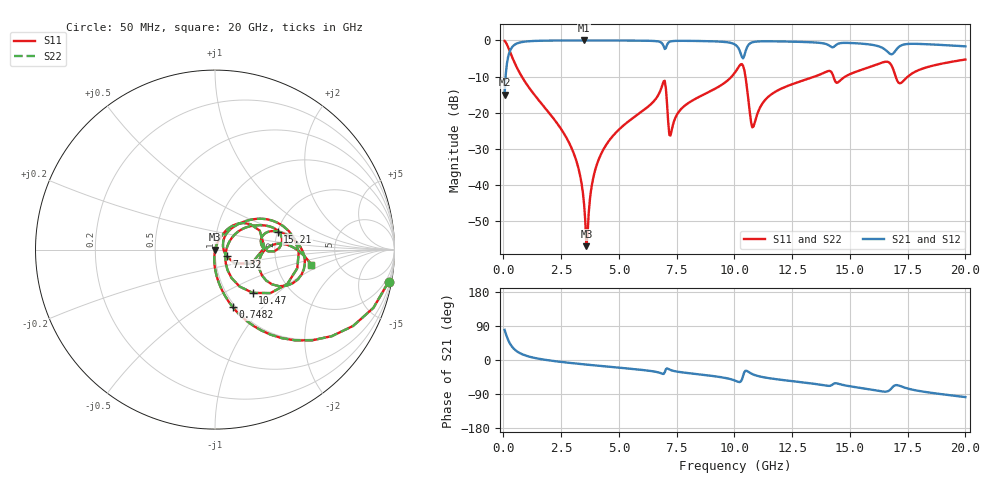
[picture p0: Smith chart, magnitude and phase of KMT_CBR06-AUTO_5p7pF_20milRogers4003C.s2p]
! Data measured by Modelithics Inc. support@modelithics.com 813-866-6335
! KEMET CBR06-AUTO 5.7pF, Pad Width= 0.851mm, Pad Length= 0.64mm, Pad Gap= 0.62mm, 20mil Rogers 4003C substrate Data, January 2022
# hz S ma R 50
! 2 Port Network Data from SP1.SP block
! freq  magS11  angS11  magS21  angS21  magS12  angS12  magS22  angS22
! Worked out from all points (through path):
!   401 points, 50 MHz to 20 GHz, reference 50 ohm
!   highest |S21| = -0.01 dB at 3.491 GHz (marker M1); lowest = -15.0 dB at 50 MHz (marker M2)
!   group delay of S21, straight-line fit = 15.2 ps
!   lowest |S11| = -57.0 dB at 3.591 GHz (marker M3), VSWR 1.00, Z = 50.1 - j0.0907 ohm
!   |S11| at or under -10 dB: 792.2 MHz to 9.883 GHz (9.091 GHz wide, 170 % of centre); 10.48 GHz to 13.48 GHz (3.003 GHz wide, 25.1 % of centre); 16.98 GHz to 17.51 GHz (531.9 MHz wide, 3.08 % of centre)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
!   |S22| runs from -57.0 to -0.1 dB; largest |S21 - S12| = 0
!   S11 on the Smith chart (normalised r, x): 50 MHz: 1, -11; 748.2 MHz: 0.97, -0.70; 7.132 GHz: 1.13, -0.09; 10.47 GHz: 1.32, -0.71; 15.21 GHz: 2.00, +0.46; 20 GHz: 3.17, -0.77
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5e7  0.984 -10.4  0.1777 79.6  0.1777 79.6  0.984 -10.4
2.99375e8  0.6763 -48.4  0.736 41.5  0.736 41.5  0.6763 -48.4
7.4825e8  0.3343 -72.9  0.9418 17.0  0.9418 17.0  0.3343 -72.9
2.74325e9  0.04386 -95.3  0.9978 -6.8  0.9978 -6.8  0.04386 -95.3
3.391625e9  0.00997 -93.9  0.9986 -10.9  0.9986 -10.9  0.00997 -93.9
3.491375e9  0.005367 -88.3  0.9986 -11.5  0.9986 -11.5  0.005367 -88.3
3.591125e9  0.001412 -39.9  0.9986 -12.1  0.9986 -12.1  0.001412 -39.9
3.94025e9  0.01472 70.7  0.9984 -14.2  0.9984 -14.2  0.01472 70.7
4.33925e9  0.03133 71.0  0.9979 -16.5  0.9979 -16.5  0.03133 71.0
6.73325e9  0.1827 50.5  0.9629 -33.1  0.9629 -33.1  0.1827 50.5
6.93275e9  0.2709 23.0  0.8362 -36.9  0.8362 -36.9  0.2709 23.0
7.13225e9  0.07484 -30.5  0.9254 -23.5  0.9254 -23.5  0.07484 -30.5
7.281875e9  0.05665 38.3  0.9751 -27.4  0.9751 -27.4  0.05665 38.3
1.0025e10  0.3598 26.5  0.8769 -54.3  0.8769 -54.3  0.3598 26.5
1.047388e10  0.3203 -48.9  0.6932 -28.6  0.6932 -28.6  0.3203 -48.9
1.0823e10  0.06373 1.5  0.9499 -38.4  0.9499 -38.4  0.06373 1.5
1.152125e10  0.1715 37.7  0.9727 -48.2  0.9727 -48.2  0.1715 37.7
1.336662e10  0.3071 26.0  0.9411 -62.1  0.9411 -62.1  0.3071 26.0
1.5212e10  0.363 16.0  0.915 -71.4  0.915 -71.4  0.363 16.0
1.670825e10  0.4914 -19.5  0.6619 -80.2  0.6619 -80.2  0.4914 -19.5
1.7207e10  0.2567 -8.5  0.8486 -69.3  0.8486 -69.3  0.2567 -8.5
2e10  0.5434 -9.1  0.8275 -97.9  0.8275 -97.9  0.5434 -9.1
